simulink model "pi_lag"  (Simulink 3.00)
settings: Solver=ode45  SolverMode=SingleTasking  StartTime=0.0  StopTime=50  MaxStep=st_size  RelTol=1e-5  AbsTol=1e-6
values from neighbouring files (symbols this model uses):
  d_through_p = get(MAIN_MENU(19),'Value')    [cback.m]    (also in imcmenu.m = 0)
  Disturb = Setpoint    [mimo_MSF1DF_sim.m]    (also in mimo_MSF2DF_sim.m)
  Satlb = temp1    [cback.m]    (also in imcmenu.m = str2num(satlbs))
  Satub = temp1    [cback.m]    (also in imcmenu.m = str2num(satubs))
  Setpoint = zeros(1,n)    [mimo_MSF1DF_sim.m]    (also in mimo_MSF2DF_sim.m)
undefined symbols (not defined in the file or in its folder): denPd, denPs, keps, numPd, numPs, Pre_fil_den, Pre_fil_num, TauX, TauY
libraries: MIMO_lib x1

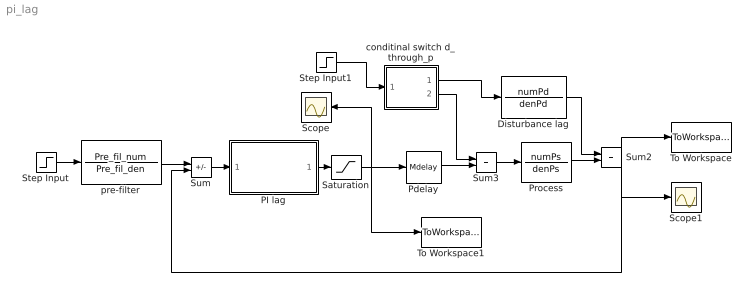
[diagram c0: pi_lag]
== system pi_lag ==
  Disturbance lag : TransferFcn  Numerator=numPd  Denominator=denPd
  PI lag : Subsystem
  Pdelay : MIMO_lib/Mdelay  Mdelay=Pdelay
  Process : TransferFcn  Numerator=numPs  Denominator=denPs
  Saturation : Saturate  UpperLimit=Satub  LowerLimit=Satlb
  Scope : Scope
  Scope1 : Scope
  Step Input : Step  Time=0  Before=0  After=Setpoint  SampleTime=0
  Step Input1 : Step  Time=0  Before=0  After=Disturb  SampleTime=0
  Sum : Sum  Inputs=+-  SaturateOnIntegerOverflow=on
  Sum2 : Sum  Inputs=++  SaturateOnIntegerOverflow=on
  Sum3 : Sum  Inputs=++  SaturateOnIntegerOverflow=on
  To Workspace : ToWorkspace  VariableName=simout  SampleTime=-1  SaveFormat=Matrix
  To Workspace1 : ToWorkspace  VariableName=effort  SampleTime=-1  SaveFormat=Matrix
  conditinal switch d_through_p : Subsystem  Description=pass input signal through out1 if condition is true.
  pre-filter : TransferFcn  Numerator=Pre_fil_num  Denominator=Pre_fil_den
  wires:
  Step Input/1 -> pre-filter/1
  pre-filter/1 -> Sum/1
  Sum/1 -> PI lag/1(In1)
  PI lag/1(Out1) -> Saturation/1
  Step Input1/1 -> conditinal switch d_through_p/1(In)
  Pdelay/1 -> Sum3/2
  conditinal switch d_through_p/2(Out1) -> Sum3/1
  conditinal switch d_through_p/1(Out2) -> Disturbance lag/1
  Sum3/1 -> Process/1
  Process/1 -> Sum2/2
  Disturbance lag/1 -> Sum2/1
  Sum2/1 -> Sum/2, To Workspace/1, Scope1/1
  Saturation/1 -> Pdelay/1, Scope/1, To Workspace1/1

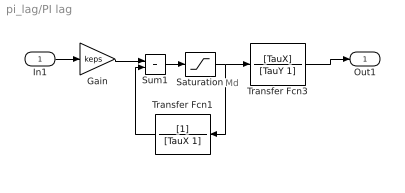
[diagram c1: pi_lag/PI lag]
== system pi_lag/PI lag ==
  note: Md
  In1 : Inport  Port=1  PortWidth=-1  SampleTime=-1  DataType=auto
  Gain : Gain  Gain=keps  SaturateOnIntegerOverflow=on
  Saturation : Saturate  UpperLimit=Satub  LowerLimit=Satlb
  Sum1 : Sum  Inputs=++  SaturateOnIntegerOverflow=on
  Transfer Fcn1 : TransferFcn  Orientation=left  Numerator=[1]  Denominator=[TauX 1]
  Transfer Fcn3 : TransferFcn  Numerator=[TauX]  Denominator=[TauY 1]
  Out1 : Outport  Port=1  InitialOutput=0
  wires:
  Transfer Fcn3/1 -> Out1/1
  Gain/1 -> Sum1/1
  In1/1 -> Gain/1
  Sum1/1 -> Saturation/1
  Saturation/1 -> Transfer Fcn3/1, Transfer Fcn1/1
  Transfer Fcn1/1 -> Sum1/2

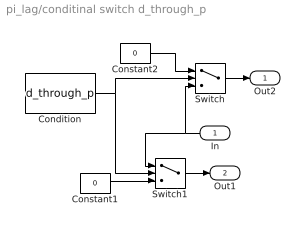
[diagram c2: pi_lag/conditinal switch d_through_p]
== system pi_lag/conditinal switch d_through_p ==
  In : Inport  Orientation=left  Port=1  PortWidth=-1  SampleTime=-1  DataType=auto
  Condition : Constant  Value=d_through_p
  Constant1 : Constant  Value=0
  Constant2 : Constant  Value=0
  Switch : Switch  Threshold=1
  Switch1 : Switch  Threshold=1
  Out2 : Outport  Port=1  InitialOutput=0
  Out1 : Outport  Port=2  InitialOutput=0
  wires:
  In/1 -> Switch/3, Switch1/1
  Condition/1 -> Switch1/2, Switch/2
  Constant1/1 -> Switch1/3
  Constant2/1 -> Switch/1
  Switch/1 -> Out2/1
  Switch1/1 -> Out1/1
